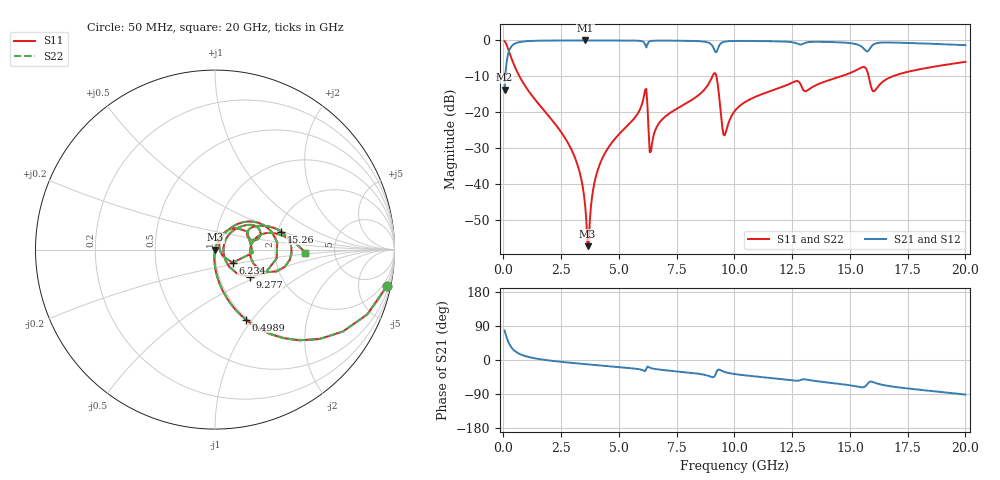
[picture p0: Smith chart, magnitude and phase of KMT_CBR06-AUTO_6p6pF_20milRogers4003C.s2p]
! Data measured by Modelithics Inc. support@modelithics.com 813-866-6335
! KEMET CBR06-AUTO 6.6pF, Pad Width= 0.851mm, Pad Length= 0.64mm, Pad Gap= 0.62mm, 20mil Rogers 4003C substrate Data, January 2022
# hz S ma R 50
! 2 Port Network Data from SP1.SP block
! freq  magS11  angS11  magS21  angS21  magS12  angS12  magS22  angS22
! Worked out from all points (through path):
!   401 points, 50 MHz to 20 GHz, reference 50 ohm
!   highest |S21| = -0.01 dB at 3.541 GHz (marker M1); lowest = -13.8 dB at 50 MHz (marker M2)
!   group delay of S21, straight-line fit = 14.1 ps
!   lowest |S11| = -57.4 dB at 3.641 GHz (marker M3), VSWR 1.00, Z = 50.1 - j0.106 ohm
!   |S11| at or under -10 dB: 692.4 MHz to 9.048 GHz (8.356 GHz wide, 172 % of centre); 9.218 GHz to 14.62 GHz (5.405 GHz wide, 45.3 % of centre); 15.81 GHz to 16.85 GHz (1.04 GHz wide, 6.36 % of centre)
!   |S22| runs from -57.4 to -0.2 dB; largest |S21 - S12| = 0
!   S11 on the Smith chart (normalised r, x): 50 MHz: 0.98, -9.43; 498.9 MHz: 0.98, -0.93; 6.234 GHz: 1.20, -0.18; 9.277 GHz: 1.39, -0.45; 15.26 GHz: 2.09, +0.49; 20 GHz: 3.01, -0.13
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5e7  0.9787 -12.0  0.2049 78.0  0.2049 78.0  0.9787 -12.0
2.495e8  0.6898 -47.1  0.7235 42.8  0.7235 42.8  0.6898 -47.1
4.98875e8  0.4256 -66.3  0.9044 23.6  0.9044 23.6  0.4256 -66.3
2.74325e9  0.03969 -95.1  0.9982 -6.4  0.9982 -6.4  0.03969 -95.1
3.391625e9  0.01074 -94.8  0.9988 -10.1  0.9988 -10.1  0.01074 -94.8
3.54125e9  0.004851 -88.8  0.9988 -10.9  0.9988 -10.9  0.004851 -88.8
3.641e9  0.001355 -51.7  0.9988 -11.4  0.9988 -11.4  0.001355 -51.7
3.990125e9  0.01222 71.6  0.9987 -13.3  0.9987 -13.3  0.01222 71.6
4.33925e9  0.02481 72.2  0.9984 -15.1  0.9984 -15.1  0.02481 72.2
6.084875e9  0.1682 45.8  0.9409 -28.4  0.9409 -28.4  0.1682 45.8
6.2345e9  0.1222 -36.7  0.8838 -17.2  0.8838 -17.2  0.1222 -36.7
6.384125e9  0.02817 31.5  0.9825 -21.3  0.9825 -21.3  0.02817 31.5
6.73325e9  0.07012 61.5  0.9932 -25.1  0.9932 -25.1  0.07012 61.5
8.877875e9  0.2473 39.3  0.9316 -41.9  0.9316 -41.9  0.2473 39.3
9.276875e9  0.2459 -38.4  0.7582 -25.9  0.7582 -25.9  0.2459 -38.4
9.576125e9  0.04745 6.3  0.9618 -31.5  0.9618 -31.5  0.04745 6.3
1.0025e10  0.1049 46.7  0.9831 -37.2  0.9831 -37.2  0.1049 46.7
1.336662e10  0.2229 30.8  0.9552 -54.2  0.9552 -54.2  0.2229 30.8
1.526188e10  0.3826 15.2  0.8885 -69.4  0.8885 -69.4  0.3826 15.2
1.605988e10  0.1969 2.5  0.8915 -59.4  0.8915 -59.4  0.1969 2.5
1.670825e10  0.3021 17.8  0.9355 -68.9  0.9355 -68.9  0.3021 17.8
2e10  0.5022 -1.9  0.8578 -91.2  0.8578 -91.2  0.5022 -1.9
